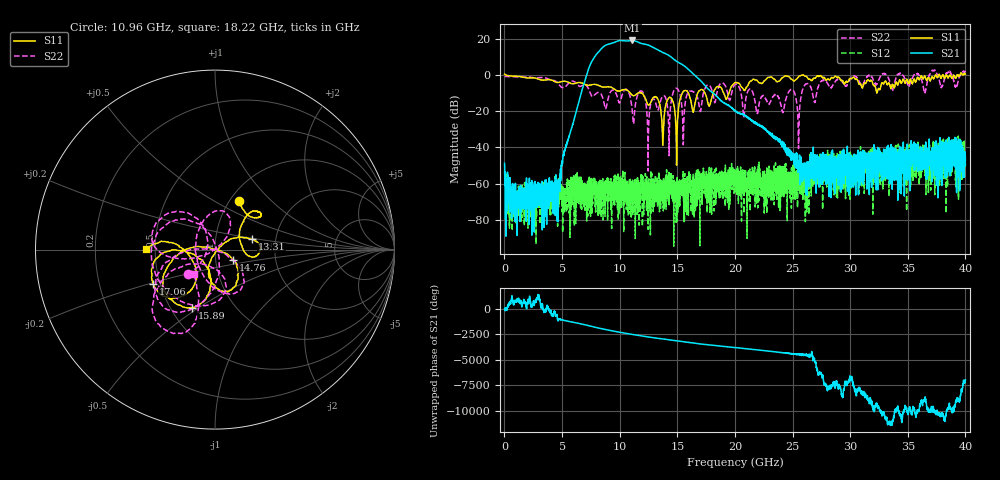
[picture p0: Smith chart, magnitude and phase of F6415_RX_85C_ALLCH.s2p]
!Keysight Technologies,N5245B,MY52451815,A.15.70.20
!Date: Wednesday, April 17, 2024 16:14:06
!Correction: S33(C  2-Port  )
!S43(C  2-Port  )
!S34(C  2-Port  )
!S44(C  2-Port  )
!S2P File: Measurements: S33, S43, S34, S44:
# Hz S  RI  R 50
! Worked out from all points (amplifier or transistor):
!   4000 points, 10 MHz to 40 GHz, reference 50 ohm
!   highest |S21| = 19.0 dB at 11.08 GHz (marker M1)
!   |S21| within 3 dB of that: 8.685 GHz to 12.65 GHz (3.964 GHz wide, 37.2 % of centre)
!   unconditionally stable (mu >= 1): 99.54 MHz to 25.86 GHz; 25.93 GHz to 32.7 GHz; 34.52 GHz to 35.53 GHz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
!   at 6.67 GHz: K = 1347.38, MAG = -6.5 dB, |S12| = -65.4 dB
!   at 20.01 GHz: K = 3731.45, MAG = -16.4 dB, |S12| = -64.6 dB
!   at 40 GHz: K = 900.72, MSG = -2.6 dB, |S12| = -44.6 dB
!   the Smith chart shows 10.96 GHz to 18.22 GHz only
!   S11 on the Smith chart (normalised r, x): 10.96 GHz: 1.10, +0.66; 13.31 GHz: 1.51, +0.18; 14.76 GHz: 1.21, -0.14; 15.89 GHz: 0.64, -0.47; 17.06 GHz: 0.46, -0.21; 18.22 GHz: 0.45, +0.00
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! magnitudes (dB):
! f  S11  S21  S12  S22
! 10 MHz  0.5  -48.7  -54.4  -0.9
! 960 MHz  -0.7  -64.4  -77.6  -1.0
! 4.44 GHz  -3.9  -72.5  -73.0  -3.4
! 6.68 GHz  -4.4  -9.4  -64.7  -6.1
! 8.35 GHz  -6.3  14.1  -71.8  -10.3
! 10.96 GHz  -10.4  19.0  -66.9  -13.8
! 11.08 GHz  -11.1  19.0  -65.0  -19.1
! 13.31 GHz  -13.4  13.8  -59.7  -19.3
! 13.34 GHz  -13.8  13.7  -63.5  -19.2
! 13.75 GHz  -37.4  12.4  -70.5  -11.6
! 14.3 GHz  -12.4  10.6  -71.7  -35.4
! 14.76 GHz  -18.9  8.3  -63.6  -8.0
! 15.52 GHz  -9.1  5.4  -59.5  -38.5
! 15.89 GHz  -9.2  3.5  -63.4  -10.3
! 17.06 GHz  -8.1  -3.4  -56.8  -18.5
! 18.22 GHz  -8.3  -10.6  -59.2  -14.8
! 20.01 GHz  -4.1  -20.1  -64.6  -5.4
! 24.96 GHz  -2.5  -44.7  -60.1  -8.3
! 25.5 GHz  -1.2  -47.8  -58.5  -31.8
! 26.67 GHz  -3.2  -52.2  -46.9  -8.5
! 33.34 GHz  -4.5  -47.0  -53.8  -2.0
! 40 GHz  0.4  -49.7  -44.6  1.5
